| IBIS file stm32h503_ufqfpn32.ibs
[IBIS ver] 4.2
[File name] stm32h503_ufqfpn32.ibs
[File Rev] 1.2
[Date] 07-05-2024
[Source] Data Created at STMicroelectronics
[Notes]  File originated from ELDO simulations.
[Disclaimer]  This information is for modeling purpose only and is
   not guaranteed. The information is subject to change without
   notice.
[Copyright] Copyright 2024 STMicroelectronics Inc.
|   Component stm32h503_ufqfpn32
[Component] stm32h503_ufqfpn32
[Manufacturer] STMicroelectronics
[Package]
| variable   typ   min   max
R_pkg  0  NA  NA
L_pkg  0  NA  NA
C_pkg  0  NA  NA
[Pin]   signal_name   model_name
1  VDD  power
2  PC14-OSC32_IN  io_ft_tamp
3  PC15-OSC32_OUT  io_ft_tamp
4  NRST  ioreset_ft_v33
5  VDDA_VREFP  nc
6  PA0  io8_ft_spi
7  PA1  io8_ft_spi
8  PA2  io8_ft_spi
9  PA3  io8_ft_spi
10  PA4  io8_ft_spi
11  PA5  io8_ft_spi
12  PA6  io8_ft_spi
13  PA7  io8_ft_spi
14  PB0  io8_ft_spi
15  PB1  io8_ft_spi
16  VCAP  nc
17  VDD  power
18  PB15  io8_ft_spi
19  PA8  io8_ft_i3c_spi
20  PA9  io8_ft_i3c_spi
21  PA11  io8usb_ft_i3c_spi_phy
22  PA12  io8usb_ft_i3c_spi_phy
23  PA13  io8_ft_i3c_spi
24  PA14  io8_ft_i3c_spi
25  PA15  io8_ft_i3c_spi
26  PB3  io8_ft_i3c_spi
27  PB4  io8_ft_i3c_spi
28  PB5  io8_ft_i3c_spi
29  PB6  io8_ft_i3c_spi
30  PB7  io8_ft_i3c_spi
31  BOOT0  io8_ft_i3c_spi
32  PB8  io8_ft_i3c_spi
0  VSS  gnd
[Package Model]   474-ufqfpn-5x5-32-240429
[Pin Mapping]   pulldown_ref   pullup_ref   | Comment
1  nc  vddio
2  gndio  vddio
3  gndio  vddio
4  gndio  vddio
5  nc  nc
6  gndio  vddio
7  gndio  vddio
8  gndio  vddio
9  gndio  vddio
10  gndio  vddio
11  gndio  vddio
12  gndio  vddio
13  gndio  vddio
14  gndio  vddio
15  gndio  vddio
16  nc  nc
17  nc  vddio
18  gndio  vddio
19  gndio  vddio
20  gndio  vddio
21  gndio  vddio
22  gndio  vddio
23  gndio  vddio
24  gndio  vddio
25  gndio  vddio
26  gndio  vddio
27  gndio  vddio
28  gndio  vddio
29  gndio  vddio
30  gndio  vddio
31  gndio  vddio
32  gndio  vddio
0  gndio  nc
|[Diff Pin]  inv_pin  vdiff  tdelay_typ  tdelay_min  tdelay_max
[Model Selector] io8_ft_i3c_spi
io8_ft_spi_ls_1v2 "GPIO SPI - 5V tolerant - low speed - 1.2V range"
io8_ft_spi_ls_1v8 "GPIO SPI - 5V tolerant - low speed - 1.8V range"
io8_ft_spi_ls_3v3 "GPIO SPI - 5V tolerant - low speed - 3.3V range"
io8_ft_spi_ms_1v2 "GPIO SPI - 5V tolerant - med speed - 1.2V range"
io8_ft_spi_ms_1v8 "GPIO SPI - 5V tolerant - med speed - 1.8V range"
io8_ft_spi_ms_3v3 "GPIO SPI - 5V tolerant - med speed - 3.3V range"
io8_ft_spi_fs_1v2 "GPIO SPI - 5V tolerant - fast speed - 1.2V range"
io8_ft_spi_fs_1v8 "GPIO SPI - 5V tolerant - fast speed - 1.8V range"
io8_ft_spi_fs_3v3 "GPIO SPI - 5V tolerant - fast speed - 3.3V range"
io8_ft_spi_hs_1v2 "GPIO SPI - 5V tolerant - high speed - 1.2V range"
io8_ft_spi_hs_1v8 "GPIO SPI - 5V tolerant - high speed - 1.8V range"
io8_ft_spi_hs_3v3 "GPIO SPI - 5V tolerant - high speed - 3.3V range"
io8_ft_hslv_spi_ls_1v2 "GPIO SPI low volt opt - 5V tolerant - low speed - 1.2V range"
io8_ft_hslv_spi_ls_1v8 "GPIO SPI low volt opt - 5V tolerant - low speed - 1.8V range"
io8_ft_hslv_spi_ls_2v5 "GPIO SPI low volt opt - 5V tolerant - low speed - 2.5V range"
io8_ft_hslv_spi_ms_1v2 "GPIO SPI low volt opt - 5V tolerant - med speed - 1.2V range"
io8_ft_hslv_spi_ms_1v8 "GPIO SPI low volt opt - 5V tolerant - med speed - 1.8V range"
io8_ft_hslv_spi_ms_2v5 "GPIO SPI low volt opt - 5V tolerant - med speed - 2.5V range"
io8_ft_hslv_spi_fs_1v2 "GPIO SPI low volt opt - 5V tolerant - fast speed - 1.2V range"
io8_ft_hslv_spi_fs_1v8 "GPIO SPI low volt opt - 5V tolerant - fast speed - 1.8V range"
io8_ft_hslv_spi_fs_2v5 "GPIO SPI low volt opt - 5V tolerant - fast speed - 2.5V range"
io8_ft_hslv_spi_hs_1v2 "GPIO SPI low volt opt - 5V tolerant - high speed - 1.2V range"
io8_ft_hslv_spi_hs_1v8 "GPIO SPI low volt opt - 5V tolerant - high speed - 1.8V range"
io8_ft_hslv_spi_hs_2v5 "GPIO SPI low volt opt - 5V tolerant - high speed - 2.5V range"
io8_ft_i3c_spi_ls_1v2 "GPIO SPI with I3C open-drain - 5V tolerant - low speed - 1.2V range"
io8_ft_i3c_spi_ls_1v8 "GPIO SPI with I3C open-drain - 5V tolerant - low speed - 1.8V range"
io8_ft_i3c_spi_ls_3v3 "GPIO SPI with I3C open-drain - 5V tolerant - low speed - 3.3V range"
io8_ft_i3c_spi_ms_1v2 "GPIO SPI with I3C open-drain - 5V tolerant - med speed - 1.2V range"
io8_ft_i3c_spi_ms_1v8 "GPIO SPI with I3C open-drain - 5V tolerant - med speed - 1.8V range"
io8_ft_i3c_spi_ms_3v3 "GPIO SPI with I3C open-drain - 5V tolerant - med speed - 3.3V range"
io8_ft_i3c_spi_fs_1v2 "GPIO SPI with I3C open-drain - 5V tolerant - fast speed - 1.2V range"
io8_ft_i3c_spi_fs_1v8 "GPIO SPI with I3C open-drain - 5V tolerant - fast speed - 1.8V range"
io8_ft_i3c_spi_fs_3v3 "GPIO SPI with I3C open-drain - 5V tolerant - fast speed - 3.3V range"
io8_ft_i3c_spi_hs_1v2 "GPIO SPI with I3C open-drain - 5V tolerant - high speed - 1.2V range"
io8_ft_i3c_spi_hs_1v8 "GPIO SPI with I3C open-drain - 5V tolerant - high speed - 1.8V range"
io8_ft_i3c_spi_hs_3v3 "GPIO SPI with I3C open-drain - 5V tolerant - high speed - 3.3V range"
io8_ft_hslv_i3c_spi_ls_1v2 "GPIO SPI low volt opt with I3C open-drain - 5V tolerant - low speed - 1.2V range"
io8_ft_hslv_i3c_spi_ls_1v8 "GPIO SPI low volt opt with I3C open-drain - 5V tolerant - low speed - 1.8V range"
io8_ft_hslv_i3c_spi_ls_2v5 "GPIO SPI low volt opt with I3C open-drain - 5V tolerant - low speed - 2.5V range"
io8_ft_hslv_i3c_spi_ms_1v2 "GPIO SPI low volt opt with I3C open-drain - 5V tolerant - med speed - 1.2V range"
io8_ft_hslv_i3c_spi_ms_1v8 "GPIO SPI low volt opt with I3C open-drain - 5V tolerant - med speed - 1.8V range"
io8_ft_hslv_i3c_spi_ms_2v5 "GPIO SPI low volt opt with I3C open-drain - 5V tolerant - med speed - 2.5V range"
io8_ft_hslv_i3c_spi_fs_1v2 "GPIO SPI low volt opt with I3C open-drain - 5V tolerant - fast speed - 1.2V range"
io8_ft_hslv_i3c_spi_fs_1v8 "GPIO SPI low volt opt with I3C open-drain - 5V tolerant - fast speed - 1.8V range"
io8_ft_hslv_i3c_spi_fs_2v5 "GPIO SPI low volt opt with I3C open-drain - 5V tolerant - fast speed - 2.5V range"
io8_ft_hslv_i3c_spi_hs_1v2 "GPIO SPI low volt opt with I3C open-drain - 5V tolerant - high speed - 1.2V range"
io8_ft_hslv_i3c_spi_hs_1v8 "GPIO SPI low volt opt with I3C open-drain - 5V tolerant - high speed - 1.8V range"
io8_ft_hslv_i3c_spi_hs_2v5 "GPIO SPI low volt opt with I3C open-drain - 5V tolerant - high speed - 2.5V range"
io8_ft_i3c_fmp_spi_3v3 "GPIO SPI with I3C fm+ open-drain - 5V tolerant - 3.3V range"
io8_ft_i3c_fmp_spi_1v8 "GPIO SPI with I3C fm+ open-drain - 5V tolerant - 1.8V range"
io8_ft_i3c_fmp_spi_1v2 "GPIO SPI with I3C fm+ open-drain - 5V tolerant - 1.2V range"
[Model Selector] io8_ft_spi
io8_ft_spi_ls_1v2 "GPIO SPI - 5V tolerant - low speed - 1.2V range"
io8_ft_spi_ls_1v8 "GPIO SPI - 5V tolerant - low speed - 1.8V range"
io8_ft_spi_ls_3v3 "GPIO SPI - 5V tolerant - low speed - 3.3V range"
io8_ft_spi_ms_1v2 "GPIO SPI- 5V tolerant - med speed - 1.2V range"
io8_ft_spi_ms_1v8 "GPIO SPI- 5V tolerant - med speed - 1.8V range"
io8_ft_spi_ms_3v3 "GPIO SPI- 5V tolerant - med speed - 3.3V range"
io8_ft_spi_fs_1v2 "GPIO SPI- 5V tolerant - fast speed - 1.2V range"
io8_ft_spi_fs_1v8 "GPIO SPI- 5V tolerant - fast speed - 1.8V range"
io8_ft_spi_fs_3v3 "GPIO SPI- 5V tolerant - fast speed - 3.3V range"
io8_ft_spi_hs_1v2 "GPIO SPI- 5V tolerant - high speed - 1.2V range"
io8_ft_spi_hs_1v8 "GPIO SPI- 5V tolerant - high speed - 1.8V range"
io8_ft_spi_hs_3v3 "GPIO SPI- 5V tolerant - high speed - 3.3V range"
io8_ft_hslv_spi_ls_1v2 "GPIO SPI low volt opt - 5V tolerant - low speed - 1.2V range"
io8_ft_hslv_spi_ls_1v8 "GPIO SPI low volt opt - 5V tolerant - low speed - 1.8V range"
io8_ft_hslv_spi_ls_2v5 "GPIO SPI low volt opt - 5V tolerant - low speed - 2.5V range"
io8_ft_hslv_spi_ms_1v2 "GPIO SPI low volt opt - 5V tolerant - med speed - 1.2V range"
io8_ft_hslv_spi_ms_1v8 "GPIO SPI low volt opt - 5V tolerant - med speed - 1.8V range"
io8_ft_hslv_spi_ms_2v5 "GPIO SPI low volt opt - 5V tolerant - med speed - 2.5V range"
io8_ft_hslv_spi_fs_1v2 "GPIO SPI low volt opt - 5V tolerant - fast speed - 1.2V range"
io8_ft_hslv_spi_fs_1v8 "GPIO SPI low volt opt - 5V tolerant - fast speed - 1.8V range"
io8_ft_hslv_spi_fs_2v5 "GPIO SPI low volt opt - 5V tolerant - fast speed - 2.5V range"
io8_ft_hslv_spi_hs_1v2 "GPIO SPI low volt opt - 5V tolerant - high speed - 1.2V range"
io8_ft_hslv_spi_hs_1v8 "GPIO SPI low volt opt - 5V tolerant - high speed - 1.8V range"
io8_ft_hslv_spi_hs_2v5 "GPIO SPI low volt opt - 5V tolerant - high speed - 2.5V range"
[Model Selector] io8usb_ft_i3c_spi_phy
io8_ft_spi_ls_1v2 "GPIO SPI - 5V tolerant - low speed - 1.2V range"
io8_ft_spi_ls_1v8 "GPIO SPI - 5V tolerant - low speed - 1.8V range"
io8_ft_spi_ls_3v3 "GPIO SPI - 5V tolerant - low speed - 3.3V range"
io8_ft_spi_ms_1v2 "GPIO SPI - 5V tolerant - med speed - 1.2V range"
io8_ft_spi_ms_1v8 "GPIO SPI - 5V tolerant - med speed - 1.8V range"
io8_ft_spi_ms_3v3 "GPIO SPI - 5V tolerant - med speed - 3.3V range"
io8_ft_spi_fs_1v2 "GPIO SPI - 5V tolerant - fast speed - 1.2V range"
io8_ft_spi_fs_1v8 "GPIO SPI - 5V tolerant - fast speed - 1.8V range"
io8_ft_spi_fs_3v3 "GPIO SPI - 5V tolerant - fast speed - 3.3V range"
io8_ft_spi_hs_1v2 "GPIO SPI - 5V tolerant - high speed - 1.2V range"
io8_ft_spi_hs_1v8 "GPIO SPI - 5V tolerant - high speed - 1.8V range"
io8_ft_spi_hs_3v3 "GPIO SPI - 5V tolerant - high speed - 3.3V range"
io8_ft_hslv_spi_ls_1v2 "GPIO SPI low volt opt - 5V tolerant - low speed - 1.2V range"
io8_ft_hslv_spi_ls_1v8 "GPIO SPI low volt opt - 5V tolerant - low speed - 1.8V range"
io8_ft_hslv_spi_ls_2v5 "GPIO SPI low volt opt - 5V tolerant - low speed - 2.5V range"
io8_ft_hslv_spi_ms_1v2 "GPIO SPI low volt opt - 5V tolerant - med speed - 1.2V range"
io8_ft_hslv_spi_ms_1v8 "GPIO SPI low volt opt - 5V tolerant - med speed - 1.8V range"
io8_ft_hslv_spi_ms_2v5 "GPIO SPI low volt opt - 5V tolerant - med speed - 2.5V range"
io8_ft_hslv_spi_fs_1v2 "GPIO SPI low volt opt - 5V tolerant - fast speed - 1.2V range"
io8_ft_hslv_spi_fs_1v8 "GPIO SPI low volt opt - 5V tolerant - fast speed - 1.8V range"
io8_ft_hslv_spi_fs_2v5 "GPIO SPI low volt opt - 5V tolerant - fast speed - 2.5V range"
io8_ft_hslv_spi_hs_1v2 "GPIO SPI low volt opt - 5V tolerant - high speed - 1.2V range"
io8_ft_hslv_spi_hs_1v8 "GPIO SPI low volt opt - 5V tolerant - high speed - 1.8V range"
io8_ft_hslv_spi_hs_2v5 "GPIO SPI low volt opt - 5V tolerant - high speed - 2.5V range"
io8_ft_i3c_spi_ls_1v2 "GPIO SPI  with I3C open-drain - 5V tolerant - low speed - 1.2V range"
io8_ft_i3c_spi_ls_1v8 "GPIO SPI  with I3C open-drain - 5V tolerant - low speed - 1.8V range"
io8_ft_i3c_spi_ls_3v3 "GPIO SPI  with I3C open-drain - 5V tolerant - low speed - 3.3V range"
io8_ft_i3c_spi_ms_1v2 "GPIO SPI  with I3C open-drain - 5V tolerant - med speed - 1.2V range"
io8_ft_i3c_spi_ms_1v8 "GPIO SPI  with I3C open-drain - 5V tolerant - med speed - 1.8V range"
io8_ft_i3c_spi_ms_3v3 "GPIO SPI  with I3C open-drain - 5V tolerant - med speed - 3.3V range"
io8_ft_i3c_spi_fs_1v2 "GPIO SPI  with I3C open-drain - 5V tolerant - fast speed - 1.2V range"
io8_ft_i3c_spi_fs_1v8 "GPIO SPI  with I3C open-drain - 5V tolerant - fast speed - 1.8V range"
io8_ft_i3c_spi_fs_3v3 "GPIO SPI  with I3C open-drain - 5V tolerant - fast speed - 3.3V range"
io8_ft_i3c_spi_hs_1v2 "GPIO SPI  with I3C open-drain - 5V tolerant - high speed - 1.2V range"
io8_ft_i3c_spi_hs_1v8 "GPIO SPI  with I3C open-drain - 5V tolerant - high speed - 1.8V range"
io8_ft_i3c_spi_hs_3v3 "GPIO SPI  with I3C open-drain - 5V tolerant - high speed - 3.3V range"
io8_ft_hslv_i3c_spi_ls_1v2 "GPIO SPI  low volt opt with I3C open-drain - 5V tolerant - low speed - 1.2V range"
io8_ft_hslv_i3c_spi_ls_1v8 "GPIO SPI  low volt opt with I3C open-drain - 5V tolerant - low speed - 1.8V range"
io8_ft_hslv_i3c_spi_ls_2v5 "GPIO SPI  low volt opt with I3C open-drain - 5V tolerant - low speed - 2.5V range"
io8_ft_hslv_i3c_spi_ms_1v2 "GPIO SPI  low volt opt with I3C open-drain - 5V tolerant - med speed - 1.2V range"
io8_ft_hslv_i3c_spi_ms_1v8 "GPIO SPI  low volt opt with I3C open-drain - 5V tolerant - med speed - 1.8V range"
io8_ft_hslv_i3c_spi_ms_2v5 "GPIO SPI  low volt opt with I3C open-drain - 5V tolerant - med speed - 2.5V range"
io8_ft_hslv_i3c_spi_fs_1v2 "GPIO SPI  low volt opt with I3C open-drain - 5V tolerant - fast speed - 1.2V range"
io8_ft_hslv_i3c_spi_fs_1v8 "GPIO SPI  low volt opt with I3C open-drain - 5V tolerant - fast speed - 1.8V range"
io8_ft_hslv_i3c_spi_fs_2v5 "GPIO SPI  low volt opt with I3C open-drain - 5V tolerant - fast speed - 2.5V range"
io8_ft_hslv_i3c_spi_hs_1v2 "GPIO SPI  low volt opt with I3C open-drain - 5V tolerant - high speed - 1.2V range"
io8_ft_hslv_i3c_spi_hs_1v8 "GPIO SPI  low volt opt with I3C open-drain - 5V tolerant - high speed - 1.8V range"
io8_ft_hslv_i3c_spi_hs_2v5 "GPIO SPI  low volt opt with I3C open-drain - 5V tolerant - high speed - 2.5V range"
io8_ft_i3c_fmp_spi_3v3 "GPIO SPI  with I3C fm+ open-drain - 5V tolerant - 3.3V range"
io8_ft_i3c_fmp_spi_1v8 "GPIO SPI  with I3C fm+ open-drain - 5V tolerant - 1.8V range"
io8_ft_i3c_fmp_spi_1v2 "GPIO SPI  with I3C fm+ open-drain - 5V tolerant - 1.2V range"
io8usb_ft_phy_ls_2v5 "USB PHY - 5V tolerant - low speed - 2.5V range"
io8usb_ft_phy_ls_3v3 "USB PHY - 5V tolerant - low speed - 3.3V range
io8usb_ft_phy_fs_2v5 "USB PHY - 5V tolerant - fast speed - 2.5V range"
io8usb_ft_phy_fs_3v3 "USB PHY - 5V tolerant - fast speed - 3.3V range"
[Model Selector] io_ft_tamp
io_ft_tamp_3v3 "IO tamper - 5V tolerant - 3.3V range"
io_ft_tamp_1v8 "IO tamper - 5V tolerant - 1.8V range"
io_ft_tamp_1v2 "IO tamper - 5V tolerant - 1.2V range"
[Model Selector] ioreset_ft_v33
ioreset_ft_v33_1v2 "Reset PAD. 5V tolerant. 1.2V range"
ioreset_ft_v33_1v8 "Reset PAD. 5V tolerant. 1.8V range"
ioreset_ft_v33_3v3 "Reset PAD. 5V tolerant. 3.3V range"
[Define Package Model]  474-ufqfpn-5x5-32-240429
[Manufacturer]  Unknown
[OEM]  Unknown
[Description]  None
[Number Of Pins]  33
[Pin Numbers]
| Pin Num   Terminal Name
31 | BOOT0
4 | NRST
6 | PA0
21 | PA11
22 | PA12
23 | PA13
24 | PA14
25 | PA15
7 | PA1
8 | PA2
9 | PA3
10 | PA4
11 | PA5
12 | PA6
13 | PA7
19 | PA8
20 | PA9
14 | PB0
18 | PB15
15 | PB1
26 | PB3
27 | PB4
28 | PB5
29 | PB6
30 | PB7
32 | PB8
2 | PC14-OSC32_IN
3 | PC15-OSC32_OUT
16 | VCAP
17 | VDD
1 | VDD
5 | VDDA_VREFP
0 | VSS
[Model Data]
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[End Model Data]
[End Package Model]
|End [Component]
| Models and submodels in the file (61): io8_ft_hslv_i3c_spi_fs_1v2 (I/O_open_drain), io8_ft_hslv_i3c_spi_fs_1v8 (I/O_open_drain), io8_ft_hslv_i3c_spi_fs_2v5 (I/O_open_drain), io8_ft_hslv_i3c_spi_hs_1v2 (I/O_open_drain), io8_ft_hslv_i3c_spi_hs_1v8 (I/O_open_drain), io8_ft_hslv_i3c_spi_hs_2v5 (I/O_open_drain), io8_ft_hslv_i3c_spi_ls_1v2 (I/O_open_drain), io8_ft_hslv_i3c_spi_ls_1v8 (I/O_open_drain), io8_ft_hslv_i3c_spi_ls_2v5 (I/O_open_drain), io8_ft_hslv_i3c_spi_ms_1v2 (I/O_open_drain), io8_ft_hslv_i3c_spi_ms_1v8 (I/O_open_drain), io8_ft_hslv_i3c_spi_ms_2v5 (I/O_open_drain), io8_ft_hslv_spi_fs_1v2 (I/O), io8_ft_hslv_spi_fs_1v8 (I/O), io8_ft_hslv_spi_fs_2v5 (I/O), io8_ft_hslv_spi_hs_1v2 (I/O), io8_ft_hslv_spi_hs_1v8 (I/O), io8_ft_hslv_spi_hs_2v5 (I/O), io8_ft_hslv_spi_ls_1v2 (I/O), io8_ft_hslv_spi_ls_1v8 (I/O), io8_ft_hslv_spi_ls_2v5 (I/O), io8_ft_hslv_spi_ms_1v2 (I/O), io8_ft_hslv_spi_ms_1v8 (I/O), io8_ft_hslv_spi_ms_2v5 (I/O), io8_ft_i3c_fmp_spi_1v2 (I/O_open_drain), io8_ft_i3c_fmp_spi_1v8 (I/O_open_drain), io8_ft_i3c_fmp_spi_3v3 (I/O_open_drain), io8_ft_i3c_spi_fs_1v2 (I/O_open_drain), io8_ft_i3c_spi_fs_1v8 (I/O_open_drain), io8_ft_i3c_spi_fs_3v3 (I/O_open_drain), io8_ft_i3c_spi_hs_1v2 (I/O_open_drain), io8_ft_i3c_spi_hs_1v8 (I/O_open_drain), io8_ft_i3c_spi_hs_3v3 (I/O_open_drain), io8_ft_i3c_spi_ls_1v2 (I/O_open_drain), io8_ft_i3c_spi_ls_1v8 (I/O_open_drain), io8_ft_i3c_spi_ls_3v3 (I/O_open_drain), io8_ft_i3c_spi_ms_1v2 (I/O_open_drain), io8_ft_i3c_spi_ms_1v8 (I/O_open_drain), io8_ft_i3c_spi_ms_3v3 (I/O_open_drain), io8_ft_spi_fs_1v2 (I/O), io8_ft_spi_fs_1v8 (I/O), io8_ft_spi_fs_3v3 (I/O), io8_ft_spi_hs_1v2 (I/O), io8_ft_spi_hs_1v8 (I/O), io8_ft_spi_hs_3v3 (I/O), io8_ft_spi_ls_1v2 (I/O), io8_ft_spi_ls_1v8 (I/O), io8_ft_spi_ls_3v3 (I/O), io8_ft_spi_ms_1v2 (I/O), io8_ft_spi_ms_1v8 (I/O), io8_ft_spi_ms_3v3 (I/O), io8usb_ft_phy_fs_2v5 (I/O), io8usb_ft_phy_fs_3v3 (I/O), io8usb_ft_phy_ls_2v5 (I/O), io8usb_ft_phy_ls_3v3 (I/O), io_ft_tamp_1v2 (I/O), io_ft_tamp_1v8 (I/O), io_ft_tamp_3v3 (I/O), ioreset_ft_v33_1v2 (I/O_open_drain), ioreset_ft_v33_1v8 (I/O_open_drain), ioreset_ft_v33_3v3 (I/O_open_drain)
